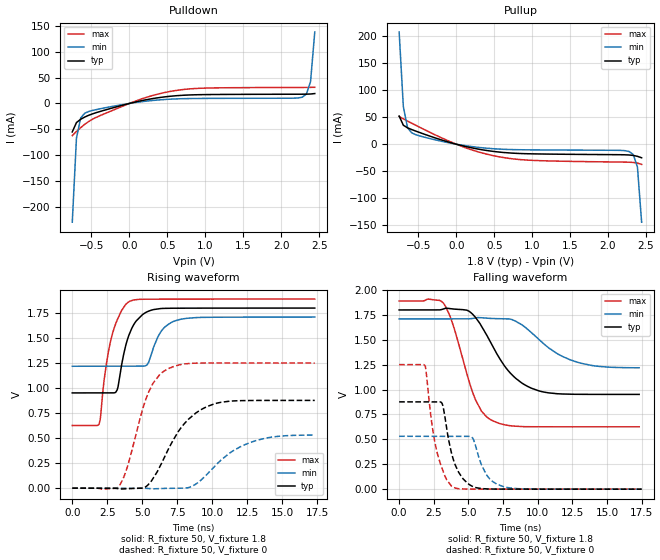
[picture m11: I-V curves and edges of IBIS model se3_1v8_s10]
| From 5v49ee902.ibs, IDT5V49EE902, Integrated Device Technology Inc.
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[Model]   se3_1v8_s10
Model_type   Output
Polarity   Non-Inverting
|   typ   min   max
C_comp   2pF   1.5pF   2.5pF
Vmeas = 0.9V
Rref = 50
Cref = 0
Vref = 0.9V
|   typ   min   max
[Voltage range]   1.8V   1.71V   1.89V
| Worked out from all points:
|   slope of the pulldown table from 0 to 0.27 V, typ, clamps not added: 32 ohm
|   slope of the pullup table from 0 to 0.27 V, typ, clamps not added: 31.6 ohm
|   rising waveform, R_fixture 50, V_fixture 1.8: 20-80 % time 977ps typ, 1.03ns min, 959ps max; typ from 0.952 V to 1.8 V
|   falling waveform, R_fixture 50, V_fixture 1.8: 20-80 % time 2.38ns typ, 2.82ns min, 1.66ns max; typ from 1.8 V to 0.952 V
|   rising waveform, R_fixture 50, V_fixture 0: 20-80 % time 2.29ns typ, 2.78ns min, 1.58ns max; typ from 0 V to 0.877 V
|   falling waveform, R_fixture 50, V_fixture 0: 20-80 % time 936ps typ, 986ps min, 916ps max; typ from 0.877 V to 0 V
[Pulldown]
|Voltage   I (typ)   I (min)   I (max)
|Note, modeling breaks down at 250mA and above.  This is well beyond the functional   |
|operating range of the device.  Should this scenario occur, catastrophic failure and   |
|possible damage to the device and/or board is of higher concern than the I-V curve   |
|behavior.  The IBIS checker will flag currents in excess of 10A with warnings.  Lines   |
|with currents in excess of 0.35 A have been commented out.  The points still remain|
|available to the user if the user desires to use them.   |
|-1.80000e+00   -2.52572e+01   -2.08112e+01   -3.26463e+01
|-1.74490e+00   -2.36799e+01   -1.95979e+01   -3.04476e+01
|-1.68980e+00   -2.21059e+01   -1.83872e+01   -2.82531e+01
|-1.63469e+00   -2.05356e+01   -1.71794e+01   -2.60635e+01
|-1.57959e+00   -1.89696e+01   -1.59750e+01   -2.38796e+01
|-1.52449e+00   -1.74087e+01   -1.47744e+01   -2.17024e+01
|-1.46939e+00   -1.58536e+01   -1.35783e+01   -1.95332e+01
|-1.41429e+00   -1.43055e+01   -1.23874e+01   -1.73739e+01
|-1.35918e+00   -1.27659e+01   -1.12027e+01   -1.52269e+01
|-1.30408e+00   -1.12368e+01   -1.00254e+01   -1.30956e+01
|-1.24898e+00   -9.72098e+00   -8.85722e+00   -1.09851e+01
|-1.19388e+00   -8.22246e+00   -7.70043e+00   -8.90351e+00
|-1.13878e+00   -6.74727e+00   -6.55830e+00   -6.86403e+00
|-1.08367e+00   -5.30512e+00   -5.43552e+00   -4.89135e+00
|-1.02857e+00   -3.91270e+00   -4.33946e+00   -3.03736e+00
|-9.73469e-01   -2.60169e+00   -3.28214e+00   -1.43100e+00
|-9.18367e-01   -1.43880e+00   -2.28475e+00   -3.94093e-01
|-8.63265e-01   -5.66865e-01   -1.38741e+00   -1.06939e-01
|-8.08163e-01   -1.52138e-01   -6.66903e-01   -7.19895e-02
-753.1mV  -54.82mA   -228.9mA   -62.01mA
-698mV    -36.89mA   -66.92mA   -54.09mA
-642.9mV  -30.52mA   -28.08mA   -46.79mA
-587.8mV  -26.13mA   -18.74mA   -40.17mA
-422.4mV  -17.04mA   -11.39mA   -25.78mA
73.47mV   2.606mA    1.636mA    4.206mA
569.4mV   14.28mA    8.482mA    23.96mA
1.01V     17.09mA    9.709mA    29.63mA
2.278V    17.85mA    12.06mA    30.89mA
2.333V    17.94mA    17.98mA    30.92mA
2.388V    18.19mA    42.4mA     30.98mA
2.443V    19.06mA    137.5mA    31.13mA
| 2.49796e+00   2.27208e-02   3.74787e-01   3.15041e-02
| 2.55306e+00   4.08756e-02   7.43068e-01   3.22551e-02
| 2.60816e+00   1.37566e-01   1.19023e+00   3.34916e-02
| 2.66327e+00   4.37820e-01   1.68221e+00   3.56718e-02
| 2.71837e+00   9.27501e-01   2.20139e+00   4.47214e-02
| 2.77347e+00   1.51885e+00   2.73835e+00   1.23384e-01
| 2.82857e+00   2.16314e+00   3.28769e+00   4.92594e-01
| 2.88367e+00   2.83803e+00   3.84607e+00   1.15125e+00
| 2.93878e+00   3.53242e+00   4.41129e+00   1.94102e+00
| 2.99388e+00   4.24015e+00   4.98190e+00   2.79125e+00
| 3.04898e+00   4.95754e+00   5.55682e+00   3.67438e+00
| 3.10408e+00   5.68219e+00   6.13525e+00   4.57781e+00
| 3.15918e+00   6.41253e+00   6.71663e+00   5.49491e+00
| 3.21429e+00   7.14740e+00   7.30048e+00   6.42176e+00
| 3.26939e+00   7.88598e+00   7.88646e+00   7.35591e+00
| 3.32449e+00   8.62763e+00   8.47428e+00   8.29574e+00
| 3.37959e+00   9.37188e+00   9.06370e+00   9.24008e+00
| 3.43469e+00   1.01184e+01   9.65453e+00   1.01881e+01
| 3.48980e+00   1.08667e+01   1.02466e+01   1.11392e+01
| 3.54490e+00   1.16168e+01   1.08398e+01   1.20928e+01
| 3.60000e+00   1.23684e+01   1.14340e+01   1.30487e+01
[Pullup]
|Voltage   I (typ)   I (min)   I (max)
|Note, modeling breaks down at 250mA and above.  This is well beyond the functional   |
|operating range of the device.  Should this scenario occur, catastrophic failure and   |
|possible damage to the device and/or board is of higher concern than the I-V curve   |
|behavior.  The IBIS checker will flag currents in excess of 10A with warnings.  Lines   |
|with currents in excess of 0.35 A have been commented out.  The points still remain|
|available to the user if the user desires to use them.   |
|-1.80000e+00   1.23492e+01   1.04530e+01   1.45809e+01
|-1.74490e+00   1.15979e+01   9.86061e+00   1.36224e+01
|-1.68980e+00   1.08480e+01   9.26940e+00   1.26656e+01
|-1.63469e+00   1.00998e+01   8.67956e+00   1.17108e+01
|-1.57959e+00   9.35349e+00   8.09124e+00   1.07584e+01
|-1.52449e+00   8.60944e+00   7.50468e+00   9.80872e+00
|-1.46939e+00   7.86800e+00   6.92013e+00   8.86233e+00
|-1.41429e+00   7.12967e+00   6.33794e+00   7.91994e+00
|-1.35918e+00   6.39506e+00   5.75851e+00   6.98248e+00
|-1.30408e+00   5.66501e+00   5.18238e+00   6.05131e+00
|-1.24898e+00   4.94068e+00   4.61027e+00   5.12833e+00
|-1.19388e+00   4.22372e+00   4.04313e+00   4.21650e+00
|-1.13878e+00   3.51650e+00   3.48228e+00   3.32063e+00
|-1.08367e+00   2.82280e+00   2.92962e+00   2.44927e+00
|-1.02857e+00   2.14888e+00   2.38803e+00   1.61954e+00
|-9.73469e-01   1.50615e+00   1.86206e+00   8.71510e-01
|-9.18367e-01   9.17564e-01   1.35944e+00   3.11233e-01
|-8.63265e-01   4.33414e-01   8.94316e-01   8.94593e-02
|-8.08163e-01   1.42396e-01   4.94089e-01   5.74619e-02
-753.1mV  52mA       207.1mA    51.2mA
-698mV    35.06mA    69.7mA     46.91mA
-642.9mV  30.25mA    30.46mA    42.81mA
-587.8mV  27.07mA    20.93mA    38.78mA
-312.2mV  13.24mA    9.215mA    19.54mA
73.47mV   -2.62mA    -1.732mA   -4.049mA
569.4mV   -14.56mA   -9.029mA   -23.39mA
1.065V    -17.95mA   -10.52mA   -30.19mA
2.278V    -19.91mA   -13.47mA   -33.25mA
2.333V    -20.75mA   -19.16mA   -33.68mA
2.388V    -22.37mA   -42.35mA   -34.85mA
2.443V    -25.08mA   -144mA     -37.25mA
| 2.49796e+00   -3.03122e-02   -4.72515e-01   -4.09753e-02
| 2.55306e+00   -4.85503e-02   -1.10341e+00   -4.57713e-02
| 2.60816e+00   -1.49867e-01   -1.94886e+00   -5.14012e-02
| 2.66327e+00   -5.72739e-01   -2.91646e+00   -5.79887e-02
| 2.71837e+00   -1.45030e+00   -3.95533e+00   -7.00790e-02
| 2.77347e+00   -2.61576e+00   -5.03908e+00   -1.50146e-01
| 2.82857e+00   -3.92793e+00   -6.15313e+00   -6.90731e-01
| 2.88367e+00   -5.32086e+00   -7.28879e+00   -1.99805e+00
| 2.93878e+00   -6.76320e+00   -8.44055e+00   -3.72340e+00
| 2.99388e+00   -8.23838e+00   -9.60470e+00   -5.63149e+00
| 3.04898e+00   -9.73678e+00   -1.07787e+01   -7.63318e+00
| 3.10408e+00   -1.12524e+01   -1.19607e+01   -9.69020e+00
| 3.15918e+00   -1.27812e+01   -1.31493e+01   -1.17833e+01
| 3.21429e+00   -1.43206e+01   -1.43434e+01   -1.39018e+01
| 3.26939e+00   -1.58683e+01   -1.55422e+01   -1.60388e+01
| 3.32449e+00   -1.74231e+01   -1.67451e+01   -1.81901e+01
| 3.37959e+00   -1.89838e+01   -1.79514e+01   -2.03526e+01
| 3.43469e+00   -2.05494e+01   -1.91609e+01   -2.25242e+01
| 3.48980e+00   -2.21193e+01   -2.03730e+01   -2.47033e+01
| 3.54490e+00   -2.36930e+01   -2.15876e+01   -2.68887e+01
| 3.60000e+00   -2.52699e+01   -2.28044e+01   -2.90795e+01
[Ramp]
|   typ   min   max
dV/dt_r   0.508/0.977n   0.294/1.029n   0.758/0.958n
dV/dt_f   0.518/2.408n   0.302/2.873n   0.769/1.679n
R_load =   50.0000
[Rising Waveform]
R_fixture = 50
V_fixture = 1.8   |Vcc_typ
V_fixture_min = 1.71 |Vcc_min
V_fixture_max = 1.89 |Vcc_max
C_fixture = 0.0p
| Time   typ   min   max
0s        951.9mV    1.218V     626.3mV
1.9ns     951.9mV    1.218V     636mV
2.377ns   951.9mV    1.218V     1.185V
2.76ns    951.9mV    1.218V     1.484V
3.236ns   994.7mV    1.218V     1.689V
4.117ns   1.553V     1.218V     1.868V
5.364ns   1.764V     1.237V     1.889V
6.317ns   1.795V     1.561V     1.889V
7.554ns   1.799V     1.682V     1.89V
17.32ns   1.8V       1.71V      1.89V
[Falling Waveform]
R_fixture = 50
V_fixture = 1.8   |Vcc_typ
V_fixture_min = 1.71 |Vcc_min
V_fixture_max = 1.89 |Vcc_max
C_fixture = 0.0p
| Time   typ   min   max
0s        1.8V       1.71V      1.89V
3.196ns   1.81V      1.71V      1.868V
3.85ns    1.81V      1.71V      1.668V
5.469ns   1.732V     1.719V     911.9mV
5.942ns   1.638V     1.722V     784mV
6.629ns   1.466V     1.715V     695.9mV
8.175ns   1.145V     1.702V     634.6mV
10.01ns   990.2mV    1.513V     626.7mV
12.94ns   952.7mV    1.272V     626.4mV
17.32ns   951.9mV    1.219V     626.4mV
[Rising Waveform]
R_fixture = 50
V_fixture = 0
C_fixture = 0.0p
| Time   typ   min   max
0s        1.215nV    7.06nV     85.21pV
3.336ns   -6.676mV   11.76nV    19mV
3.899ns   -4.969mV   -30.39nV   197.2mV
5.403ns   31.73mV    -3.007mV   943.3mV
6.766ns   362.1mV    -1.95mV    1.188V
8.286ns   687mV      4.692mV    1.245V
10ns      836mV      192.8mV    1.251V
11.36ns   870.6mV    361.4mV    1.251V
12.94ns   876.4mV    467mV      1.251V
17.32ns   876.9mV    530.7mV    1.251V
[Falling Waveform]
R_fixture = 50
V_fixture = 0
C_fixture = 0.0p
| Time   typ   min   max
0s        876.9mV    531.2mV    1.251V
1.899ns   876.9mV    531.2mV    1.229V
2.382ns   876.9mV    531.2mV    637.1mV
2.69ns    876.9mV    531.2mV    397.9mV
3.174ns   829.6mV    531.2mV    179.9mV
3.897ns   303.8mV    531.2mV    19.98mV
5.262ns   30.29mV    520mV      640.6uV
6.25ns    2.702mV    156.2mV    437.5uV
7.5ns     723.8uV    26.03mV    291.7uV
17.5ns    44.12uV    89.5uV     23.37uV
